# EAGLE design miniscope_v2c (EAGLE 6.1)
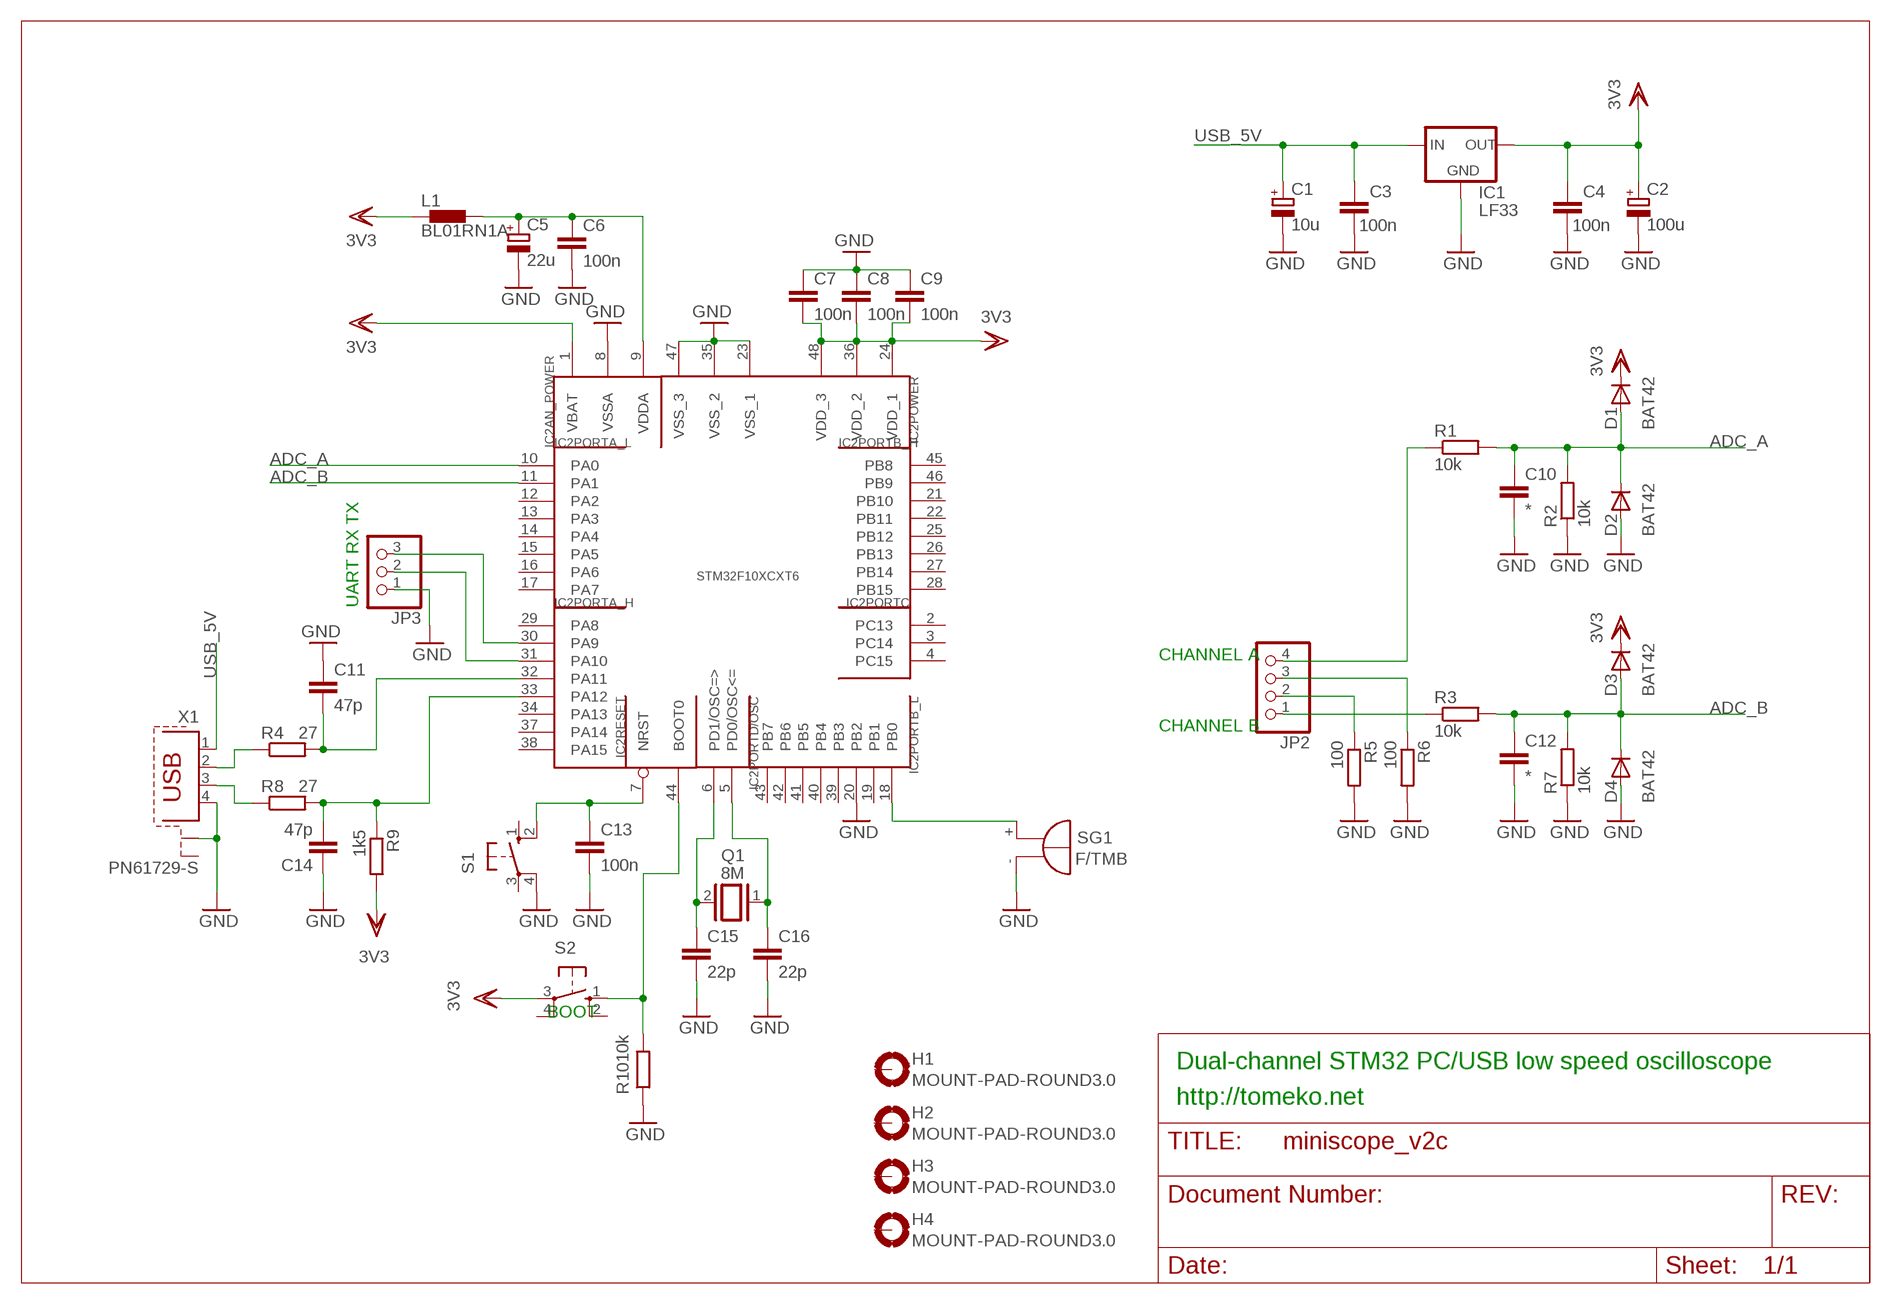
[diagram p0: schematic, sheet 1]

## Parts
C1  10u  CPOL-EUE2.5-5  [E2,5-5]
C2  100u  CPOL-EUE2.5-6  [E2,5-6]
C3  100n  C-EUC0805K  [C0805K]
C4  100n  C-EUC0805K  [C0805K]
C5  22u  CPOL-EUE2.5-5  [E2,5-5]
C6  100n  C-EUC0805K  [C0805K]
C7  100n  C-EUC0805K  [C0805K]
C8  100n  C-EUC0805K  [C0805K]
C9  100n  C-EUC0805K  [C0805K]
C10  *  C-EUC0805K  [C0805K]
C11  47p  C-EUC0805K  [C0805K]
C12  *  C-EUC0805K  [C0805K]
C13  100n  C-EUC0805K  [C0805K]
C14  47p  C-EUC0805K  [C0805K]
C15  22p  C-EUC0805K  [C0805K]
C16  22p  C-EUC0805K  [C0805K]
D1  BAT42  1N4148DO35-7  [DO35-7]
D2  BAT42  1N4148DO35-7  [DO35-7]
D3  BAT42  1N4148DO35-7  [DO35-7]
D4  BAT42  1N4148DO35-7  [DO35-7]
H1  MOUNT-PAD-ROUND3.0  [3,0-PAD]
H2  MOUNT-PAD-ROUND3.0  [3,0-PAD]
H3  MOUNT-PAD-ROUND3.0  [3,0-PAD]
H4  MOUNT-PAD-ROUND3.0  [3,0-PAD]
IC1  LF33  LFXXCV  [DPACK_1]
IC2  STM32F10XCXT6  [TQFP48]
JP2  PINHD-1X4  [1X04]
JP3  PINHD-1X3  [1X03]
L1  BL01RN1A  [BL01RN1A]
Q1  8M  XTAL/S  [QS]
R1  10k  R-R0805  [R0805]
R2  10k  R-R0805  [R0805]
R3  10k  R-R0805  [R0805]
R4  27  R-R0805  [R0805]
R5  100  R-R0805  [R0805]
R6  100  R-R0805  [R0805]
R7  10k  R-R0805  [R0805]
R8  27  R-R0805  [R0805]
R9  1k5  R-R0805  [R0805]
R10  10k  R-R0805  [R0805]
S1  10-XX  [B3F-10XX]
S2  10-XX  [B3F-10XX]
SG1  F/TMB  [F/TMB]
X1  PN61729-S  [PN61729-S]

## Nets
ADC_A: C10.1 D1.A D2.C IC2.10(PORTA_L:PA0) R1.2 R2.2
ADC_B: C12.1 D3.A D4.C IC2.11(PORTA_L:PA1) R3.2 R7.2
GND: C1.- C2.- C3.1 C4.1 C5.- C6.2 C7.1 C8.1 C9.1 C10.2 C11.1 C12.2 C13.2 C14.1 C15.2 C16.2 D2.A D4.A IC1.C(GND) IC2.8(AN_POWER:VSSA) IC2.20(PORTB_L:PB2) IC2.23(POWER:VSS_1) IC2.35(POWER:VSS_2) IC2.47(POWER:VSS_3) JP3.1 R2.1 R5.2 R6.2 R7.1 R10.1 S1.4(P1) SG1.- X1.4 X1.S1
N$1: IC2.44(RESET:BOOT0) R10.2 S2.1(S)
N$2: C5.+ C6.1 IC2.9(AN_POWER:VDDA) L1.2
N$3: JP2.2 R5.1
N$4: C13.1 IC2.7(RESET:NRST) S1.2(S1)
N$5: R4.1 X1.2
N$6: R8.1 X1.3
N$7: C14.2 IC2.33(PORTA_H:PA12) R8.2 R9.1
N$8: C11.2 IC2.32(PORTA_H:PA11) R4.2
N$9: IC2.31(PORTA_H:PA10) JP3.2
N$10: JP2.3 R6.1
N$11: JP2.4 R1.1
N$12: JP2.1 R3.1
N$14: C16.1 IC2.5(PORTD/OSC:PD0/OSC<=) Q1.1
N$15: IC2.18(PORTB_L:PB0) SG1.+
N$16: IC2.30(PORTA_H:PA9) JP3.3
N$37: C15.1 IC2.6(PORTD/OSC:PD1/OSC=>) Q1.2
USB_5V: C1.+ C3.2 IC1.B(IN) X1.1
VDD: C2.+ C4.2 C7.2 C8.2 C9.2 D1.C D3.C IC1.E(OUT) IC2.1(AN_POWER:VBAT) IC2.24(POWER:VDD_1) IC2.36(POWER:VDD_2) IC2.48(POWER:VDD_3) L1.1 R9.2 S2.3(P) ; supply symbol labelled 3V3
Unconnected: H1.B3,0(MOUNT) H2.B3,0(MOUNT) H3.B3,0(MOUNT) H4.B3,0(MOUNT) IC2.2(PORTC:PC13) IC2.3(PORTC:PC14) IC2.4(PORTC:PC15) IC2.12(PORTA_L:PA2) IC2.13(PORTA_L:PA3) IC2.14(PORTA_L:PA4) IC2.15(PORTA_L:PA5) IC2.16(PORTA_L:PA6) IC2.17(PORTA_L:PA7) IC2.19(PORTB_L:PB1) IC2.21(PORTB_H:PB10) IC2.22(PORTB_H:PB11) IC2.25(PORTB_H:PB12) IC2.26(PORTB_H:PB13) IC2.27(PORTB_H:PB14) IC2.28(PORTB_H:PB15) IC2.29(PORTA_H:PA8) IC2.34(PORTA_H:PA13) IC2.37(PORTA_H:PA14) IC2.38(PORTA_H:PA15) IC2.39(PORTB_L:PB3) IC2.40(PORTB_L:PB4) IC2.41(PORTB_L:PB5) IC2.42(PORTB_L:PB6) IC2.43(PORTB_L:PB7) IC2.45(PORTB_H:PB8) IC2.46(PORTB_H:PB9) S1.1(S) S1.3(P) S2.2(S1) S2.4(P1) X1.S2

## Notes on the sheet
- UART RX TX
- CHANNEL A
- CHANNEL B
- BOOT
- Dual-channel STM32 PC/USB low speed oscilloscope
- http://tomeko.net

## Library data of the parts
C1 C2 C5 = resistor:CPOL-EU: POLARIZED CAPACITOR, European symbol
C3 C4 C6-C16 = resistor:C-EU: CAPACITOR, European symbol
D1-D4 = diode:1N4148: DIODE
H1-H4 = holes:MOUNT-PAD-ROUND: MOUNTING PAD, round
IC1 = lf33:LFXXCV: VOLTAGE REGULATOR
IC2 = stm32:STM32F10XCXT6: ST STM32F101/103 48pin LQFP
JP2 = pinhead:PINHD-1X4: PIN HEADER
JP3 = pinhead:PINHD-1X3: PIN HEADER
L1 = inductors:BL0: Noise Suppression Products/EMI Suppression Filters, Lead EMIFIL(R) Inductor Type
Q1 = special:XTAL/S: CRYSTAL
R1-R10 = quantum-sensor:R: Resistor
S1 S2 = switch-omron:10-XX: OMRON SWITCH; MPN: B3F-1000; OC_FARNELL: 176432; OC_NEWARK: 36M3542
SG1 = buzzer:F/TMB: BUZZER; OC_FARNELL: unknown; OC_NEWARK: unknown
X1 = con-berg:PN61729-S: BERG USB connector; OC_FARNELL: unknown; OC_NEWARK: unknown

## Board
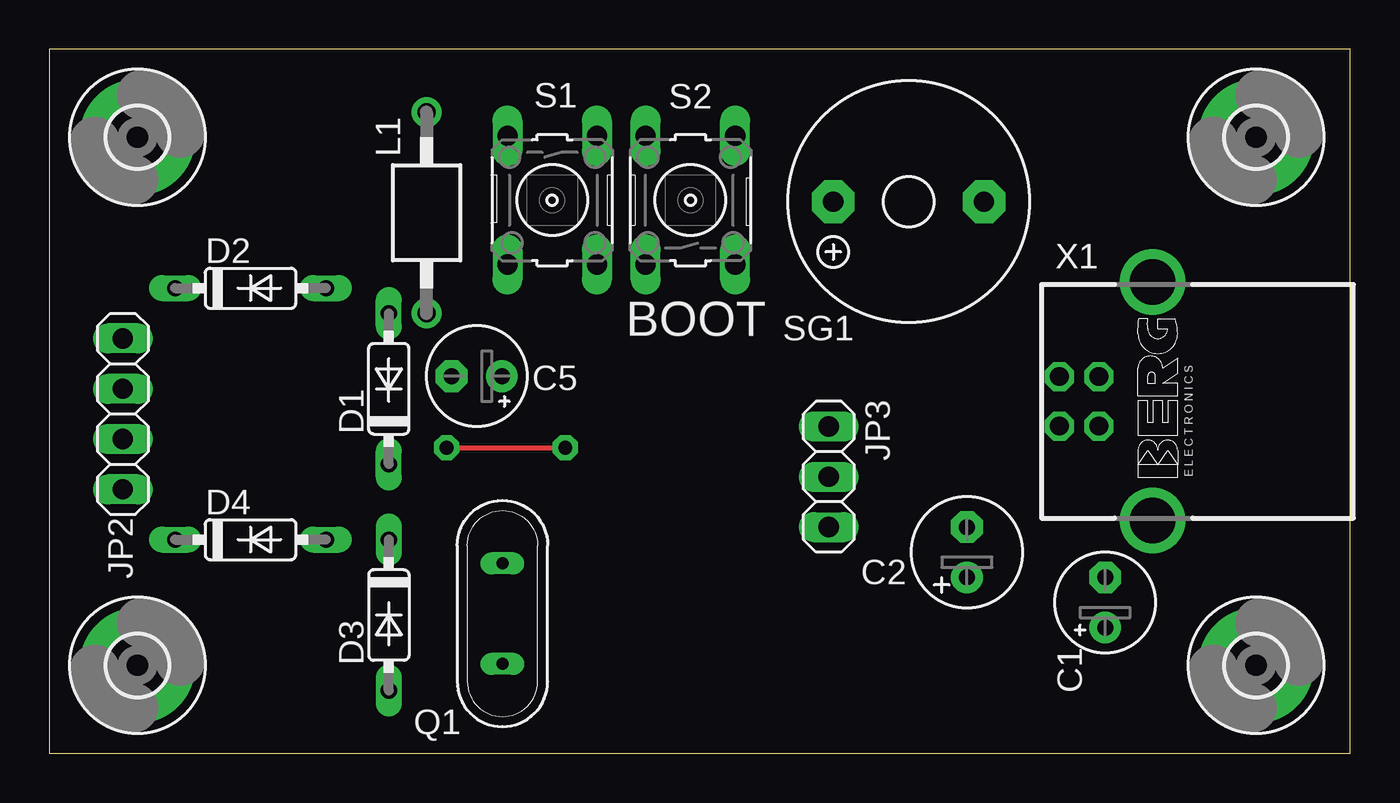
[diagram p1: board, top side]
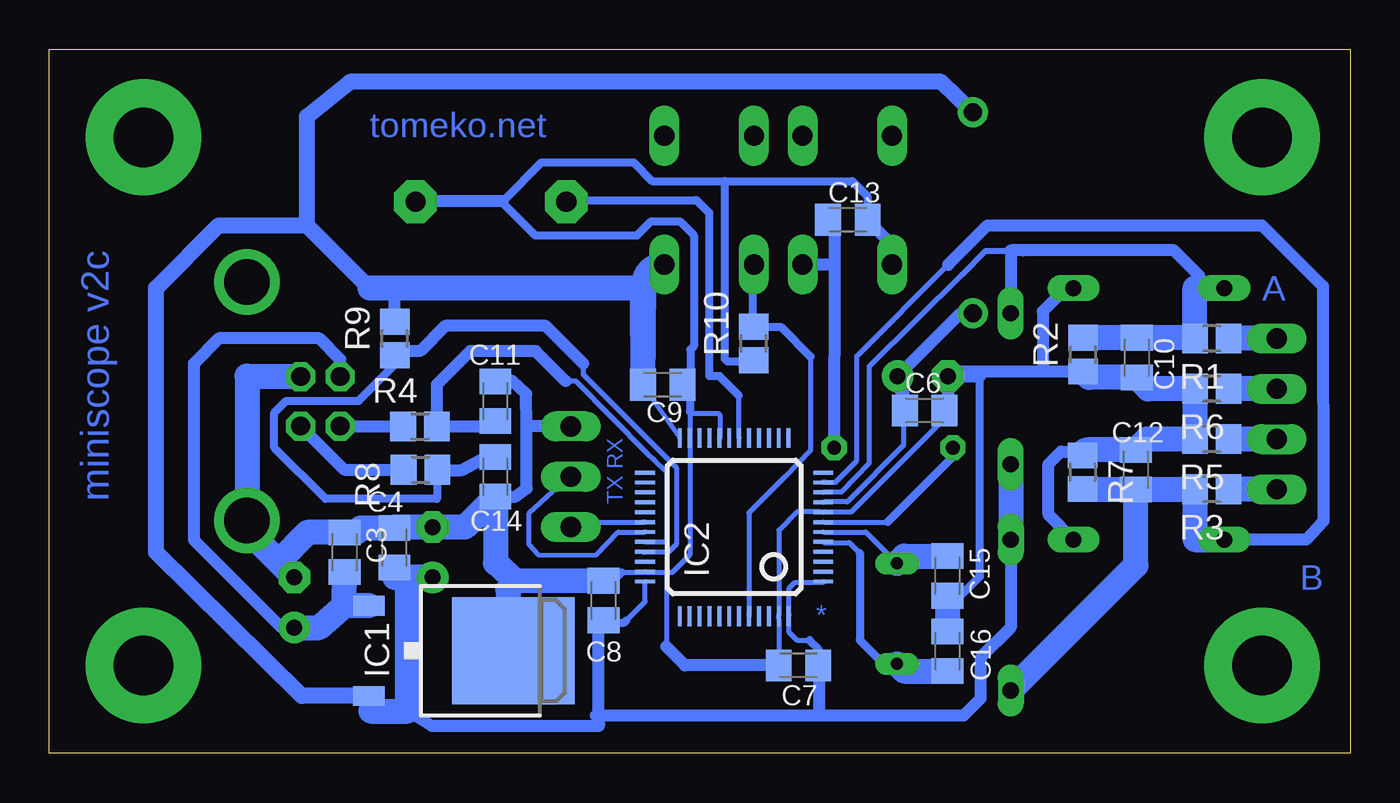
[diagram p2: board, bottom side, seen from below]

Size 65.71 x 35.55 mm. Coordinates in mm from the lower left corner, seen from the top.
Outline: 0,0 65.71,0 65.71,35.55 0,35.55 0,0
Copper layers (1*16): Top 0.035mm / dielectric 1.5mm / Bottom 0.035mm
Design rules: minimum track width 10mil, minimum drill 24mil, track to track 8mil, track to pad 8mil, pad to pad 8mil, via to via 8mil, smd to smd 8mil, copper to edge 40mil, drill to drill 8mil, minimum pad ring 10mil, minimum via ring 8mil, stop-mask expansion 4mil, vias tented up to drill 0mil, thermal gap 10mil

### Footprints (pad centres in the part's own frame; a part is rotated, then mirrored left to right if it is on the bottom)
E2,5-5 = drill 0.813 pad 1.6: + -1.27,0 | drill 0.813 pad 1.6 octagon: - 1.27,0
E2,5-6 = drill 0.813 pad 1.6: + -1.27,0 | drill 0.813 pad 1.6 octagon: - 1.27,0
C0805K = smd 1.3 x 1.6: 1 -1,0; 2 1,0
DO35-7 = drill 0.813 long: A 3.81,0; C -3.81,0
3,0-PAD = drill 3 pad 5.842: B3,0 0,0
DPACK_1 = smd 1 x 1.6: B -2.28,-4.8; E 2.28,-4.8 | smd 5.4 x 6.2: C 0,2.5
TQFP48 = smd 0.2 x 1: 1 -2.75,-4.5; 2 -2.25,-4.5; 3 -1.75,-4.5; 4 -1.25,-4.5; 5 -0.75,-4.5; 6 -0.25,-4.5; 7 0.25,-4.5; 8 0.75,-4.5; 9 1.25,-4.5; 10 1.75,-4.5; 11 2.25,-4.5; 12 2.75,-4.5; 25 2.75,4.5; 26 2.25,4.5; 27 1.75,4.5; 28 1.25,4.5; 29 0.75,4.5; 30 0.25,4.5; 31 -0.25,4.5; 32 -0.75,4.5; 33 -1.25,4.5; 34 -1.75,4.5; 35 -2.25,4.5; 36 -2.75,4.5 | smd 1 x 0.2: 13 4.5,-2.75; 14 4.5,-2.25; 15 4.5,-1.75; 16 4.5,-1.25; 17 4.5,-0.75; 18 4.5,-0.25; 19 4.5,0.25; 20 4.5,0.75; 21 4.5,1.25; 22 4.5,1.75; 23 4.5,2.25; 24 4.5,2.75; 37 -4.5,2.75; 38 -4.5,2.25; 39 -4.5,1.75; 40 -4.5,1.25; 41 -4.5,0.75; 42 -4.5,0.25; 43 -4.5,-0.25; 44 -4.5,-0.75; 45 -4.5,-1.25; 46 -4.5,-1.75; 47 -4.5,-2.25; 48 -4.5,-2.75
1X04 = drill 1.016 long: 1 -3.81,0; 2 -1.27,0; 3 1.27,0; 4 3.81,0
1X03 = drill 1.016 long: 1 -2.54,0; 2 0,0; 3 2.54,0
BL01RN1A = drill 0.9 pad 1.5: 1 -5.08,0; 2 5.08,0
QS = drill 0.61 long: 1 -2.54,0; 2 2.54,0
R0805 = smd 1.3 x 1.5: 1 -0.85,0; 2 0.85,0
B3F-10XX = drill 1.016 long: 1 -3.251,2.261; 2 3.251,2.261; 3 -3.251,-2.261; 4 3.251,-2.261
F/TMB = drill 1.016 pad 2.159 octagon: + 3.81,0; - -3.81,0
PN61729-S = drill 0.95 octagon: 1 1.25,4.71; 2 -1.25,4.71; 3 -1.25,2.71; 4 1.25,2.71 | drill 2.3 pad 2.9: S1 -6.02,0; S2 6.02,0

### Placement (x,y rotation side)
C1  53.34,7.62 90 top
C2  46.35,10.16 90 top
C3  50.8,10.16 270 bottom
C4  48.29,10.39 270 bottom
C5  21.59,19.05 180 top
C6  21.49,17.32 0 bottom
C7  27.86,4.45 0 bottom
C8  37.72,7.72 270 bottom
C9  34.72,18.62 180 bottom
C10  10.77,19.99 270 bottom
C11  43.18,17.78 270 bottom
C12  10.82,14.33 90 bottom
C13  25.37,26.95 0 bottom
C14  43.18,13.97 90 bottom
C15  20.35,8.97 270 bottom
C16  20.35,5.16 90 bottom
D1  17.14,18.41 90 top
D2  10.16,23.5 0 top
D3  17.14,6.99 270 top
D4  10.16,10.79 0 top
H1  60.96,4.45 0 top
H2  60.96,31.11 0 top
H3  4.45,31.11 0 top
H4  4.45,4.45 0 top
IC1  44.78,5.18 270 bottom
IC2  31.11,11.43 90 bottom
JP2  3.71,17.14 90 top
JP3  39.37,13.97 270 top
L1  19.05,27.3 270 top
Q1  22.89,7.06 90 top
R1  6.99,20.95 180 bottom
R2  13.49,20.14 90 bottom
R3  6.99,13.34 180 bottom
R4  46.99,16.51 0 bottom
R5  6.99,15.88 180 bottom
R6  6.99,18.41 180 bottom
R7  13.51,14.2 270 bottom
R8  46.96,14.33 0 bottom
R9  48.26,20.95 90 bottom
R10  30.12,20.7 90 bottom
S1  25.4,27.94 270 top
S2  32.38,27.94 90 top
SG1  43.41,27.86 180 top
X1  55.73,17.78 90 top

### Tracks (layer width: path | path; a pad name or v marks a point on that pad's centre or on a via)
ADC_A
  Bottom 0.254: 19.61,24.18 24.28,19.56 24.28,14.66 25.68,13.21 26.52,13.21 IC2.10 | 17.17,22.25 D1.A
  Bottom 0.305: 19.61,24.18 18.41,25.38 | 18.41,25.38 17.14,25.4 | 18.41,25.38 16.51,25.38
  Bottom 0.406: 16.51,25.38 16.51,25.4
  Bottom 0.61: 7.62,23.5 7.62,24.13 8.89,25.4 16.51,25.4 17.14,25.4 D1.A | 17.17,22.25 17.14,22.28
  Bottom 1.27: D2.C 7.62,23.5 7.83,23.5 R1.2 7.87,20.99 C10.1 R2.2 13.49,20.95 13.34,20.95
ADC_B
  Bottom 0.254: 20.31,24.68 24.92,20.07 24.92,14.78 26.01,13.69 26.49,13.69 26.52,13.72 26.62,13.72 IC2.11 | R3.2 7.82,13.31 8.26,13.34
  Bottom 0.61: 20.3,24.69 20.31,24.68 18.31,26.67 4.45,26.67 1.37,23.6 1.35,11.73 2.21,10.79 D4.C
  Bottom 1.27: C12.1 8.26,13.34 | R3.2 7.83,10.79 D4.C | C12.1 13.49,13.33 R7.2 | D3.A 10.82,9.5 C12.1
GND
  Bottom 0.254: 19.79,7.92 C15.2 19.68,7.95 | 33.25,17.17 31.93,17.17 31.83,17.07 31.83,15.95 IC2.20 | 33.35,17.27 33.25,17.17 | 33.35,18.59 C9.1 | 33.25,17.17 33.35,17.17 33.35,15.95 IC2.23 33.33,15.85 33.33,10.06 34.24,9.14 34.54,9.14 | 36.8,9.14 35.69,9.14 IC2.35 35.56,9.14 34.54,9.14 | C8.1 37.92,8.64 38.1,8.46 38.1,8.26 37.69,8.26 | 13.59,15.09 R7.1 | 34.54,9.14 34.54,5.38 | 28.85,4.37 C7.1 28.85,4.47 28.85,6.81 IC2.47 28.85,7.01 28.85,11.28 27.94,12.19 26.72,12.19 IC2.8 26.52,12.19 25.2,12.19 20.55,16.84 20.55,17.17 20.57,17.14 C6.2 | 55.73,12.29 55.78,12.29 X1.S1 | 42.55,4.47 42.57,4.47 IC1.C | 47.85,11.43 47.85,11.48 C4.1 | 14.02,23.47 D2.A | 31.6,19.91 31.5,19.81 | 30.18,19.81 R10.1 | 33.33,18.69 C9.1 | 47.17,27.89 SG1.- | 42.8,27.79 42.8,27.89 | 33.33,18.8 C9.1
  Bottom 0.406: 33.35,18.59 33.35,17.27 | 31.5,19.81 30.18,19.81 | 36.8,9.14 37.69,8.26 | 42.8,27.89 40.84,29.84 36.2,29.84 35.26,28.91 31.6,28.91 | 42.8,27.79 41.17,26.16 36.02,26.16 35.31,26.87 33.86,26.87 33.15,26.16 33.15,20.57 33.33,20.4 33.33,18.8 33.33,18.64 | 19.68,7.95 18.69,8.94 18.69,19.05 | 31.6,28.91 31.6,19.91 | 31.6,28.91 25.15,28.91 24.38,28.14 24.38,27 24.41,26.98 24.4,26.98 C13.2
  Bottom 0.61: C14.1 42.17,12.97 41.6,13.39 41.6,16.51 | 41.6,16.51 41.63,18.16 42.32,18.8 43.18,19.05 C11.1 | JP3.1 41.6,16.51 | 28.85,4.37 C7.1 33.6,4.45 34.54,5.38 | D4.A 15.24,12.06 15.24,14.61 14.61,15.24 13.34,15.24 13.51,15.06 R7.1 | 42.8,27.89 47.17,27.89 | C5.- 18.69,19.05 | C5.- 20.08,19.29 15.37,19.29 | 15.37,19.29 R2.1 13.34,19.14 13.34,19.05 | D2.A 14.35,23.5 15.52,22.33 15.52,19.45 15.37,19.29 | C5.- 20.32,17.41 C6.2 20.32,17.14 | S1.4 23.14,25.68 24.38,26.91 C13.2
  Bottom 1.27: R2.1 13.19,18.99 C10.2 10.2,18.41 R6.2 R5.2 10.27,15.88 C12.2 13.24,15.33 arc-90 R7.1 | C16.2 C15.2 arc90 20.32,7.94 20.32,7.62 | 55.73,11.91 55.73,12.29 55.73,19.05 55.71,19.03 X1.4 | X1.S1 55.73,11.28 54.14,9.69 | 54.14,9.69 C1.- | 54.14,9.69 52.67,11.16 C3.1 50.19,11.18 49.98,11.39 C4.1 | 48.26,11.43 47.85,11.43 C2.- 44.72,11.43 C14.1 43.18,9.62 42.16,8.7 | C8.1 42.16,8.7 | 42.16,8.7 42.55,8.26 42.55,4.47 42.55,4.45
N$1
  Bottom 0.254: 27.25,20.04 27.25,15.32 28.55,13.97 30.38,12.14 30.38,7.01 IC2.44 | 30.07,21.54 R10.2 30.18,21.64 | 30.18,24.69 S2.1
  Bottom 0.406: 27.25,20.04 28.75,21.54 30.07,21.54 | 30.18,21.64 30.18,24.69
N$2
  Bottom 0.254: IC2.9 26.52,12.7 25.4,12.7 22.55,15.57 22.55,16.66 C6.1 22.55,16.76 | 19.1,22.35 19.1,22.86 L1.2 | C5.+ 22.86,18.59
  Bottom 0.61: 22.55,16.76 22.55,18.19 22.76,18.39 C5.+ 19.68,22.23 L1.2
N$3
  Bottom 1.27: JP2.2 R5.1
N$4  (via drill 0.7 pad 1.27)
  Top 0.254: v20.07,15.44 v26.06,15.44
  Bottom 0.254: IC2.7 23.37,11.68
  Bottom 0.406: 23.37,11.68 20.07,14.99 v20.07,15.44
  Bottom 0.61: v26.06,15.44 26.04,24.69 | 26.04,24.69 S1.2 | 26.04,24.69 26.04,26.61 C13.1
N$5
  Bottom 0.254: R4.1 47.85,16.56 47.62,16.53
  Bottom 0.61: X1.2 47.62,16.53 47.62,16.51
N$6
  Bottom 0.61: X1.3 50.81,14.33 R8.1
N$7
  Bottom 0.254: 35.69,10.13 IC2.33 35.56,10.16 34.44,10.16 34.04,10.57 34.04,14.43 38.73,19.13 38.73,19.68 | C14.2 43.18,14.94 43.31,15.17 | 48.26,20.12 R9.1 48.36,20.12 | 46.13,14.02 R8.2
  Bottom 0.406: 46.13,14.02 46.13,12.85 51.77,12.85 54.36,15.44 54.36,17.2 53.75,17.8 50.09,17.8 48.26,19.63 R9.1
  Bottom 0.61: R8.2 46.12,14.3 44.88,14.3 43.31,15.17 43.18,15.24 | 38.73,19.68 40.64,21.59 45.72,21.59 46.99,20.32 48.26,20.32 48.26,20.12
N$8
  Bottom 0.254: IC2.32 35.56,10.67 34.65,10.67 34.54,10.77 34.54,14.22 35.15,14.83 35.53,15.19 39.12,18.8 39.62,18.8 | 46.13,16.76 R4.2
  Bottom 0.61: C11.2 43.18,16.51 R4.2 46.14,18.63 44.45,20.32 41.15,20.32 39.62,18.8
N$9
  Bottom 0.254: IC2.31 35.66,11.18 36.98,11.18 38.1,10.01 41.02,10.03 41.5,10.57 41.5,12.09 39.42,14.02 JP3.2
N$10
  Bottom 1.27: JP2.3 R6.1
N$11
  Bottom 1.27: JP2.4 R1.1
N$12
  Bottom 1.27: JP2.1 R3.1
N$14
  Bottom 0.254: IC2.5 26.58,10.64 25.3,10.64 24.77,10.11
  Bottom 0.406: 24.77,10.11 24.77,5.71 23.57,4.52 Q1.1
  Bottom 1.27: Q1.1 22.52,4.16 C16.1
N$15
  Bottom 0.254: 30.89,18.09 30.89,15.95 IC2.18 | SG1.+ 39.62,27.84 39.52,27.84
  Bottom 0.406: 39.52,27.84 39.42,27.94 33.02,27.94 32.38,27.3 32.38,19.05 31.85,19.05 30.89,18.09
N$16
  Bottom 0.254: 39.12,11.68 JP3.3 39.01,11.68 35.76,11.68 IC2.30 35.66,11.68
N$37
  Bottom 0.254: IC2.6 24.46,11.18 Q1.2 | Q1.2 22.86,9.58 22.86,9.53 22.89,9.55 Q1.2
  Bottom 1.27: Q1.2 22.52,9.97 C15.1
USB_5V
  Bottom 0.61: X1.1 51.02,19.9 52.07,20.95 57.15,20.95 58.42,19.68 58.42,10.79 53.98,6.35 C1.+
  Bottom 1.27: IC1.B 50.83,7.46 | 50.83,7.46 C3.2 | C1.+ 52.09,6.35 50.83,7.46
VDD
  Bottom 0.254: 27.3,5.71 27.94,5.71 28.37,6.15 28.37,6.92 IC2.48 28.35,7.01 28.35,8.33 28.04,8.64 26.62,8.64 IC2.1 | 37.9,6.6 C8.2 38,6.6 | 48.36,21.84 R9.2 | 26.82,4.37 C7.2 | 52.53,27.03 52.7,26.67 | 49.48,2.13 IC1.E | 17.17,10.87 D3.C | 17.17,14.53 D1.C | IC2.24 35.75,18.62 | 36.58,6.71 35.62,7.67 IC2.36
  Bottom 0.406: 27.3,5.71 26.86,5.27 C7.2 | 36.58,6.71 36.68,6.6 37.9,6.6
  Bottom 0.61: 38,6.6 38,1.91 | 38,1.91 37.95,1.37 46.38,1.37 47.62,2.13 | 26.82,4.37 26.82,1.91 | 26.82,1.91 38,1.91 | 38.1,1.91 38,1.91 | 17.17,10.87 17.14,10.85 17.14,6.35 18.67,4.83 18.67,2.77 19.53,1.91 26.82,1.91 | 48.26,22.23 48.26,23.5
  Bottom 0.813: IC1.E 52.97,2.9 60.33,10.16 60.33,23.5 57.15,26.67 52.7,26.67 | 52.7,26.67 49.53,23.5 | 48.26,22.23 R9.2 48.26,21.59 | L1.1 20.65,33.91 50.52,33.91 52.7,32.16 52.7,26.67
  Bottom 1.27: C2.+ 47.62,8.89 | 49.48,2.13 47.62,2.13 47.62,8.89 | 47.62,8.89 48.26,8.89 C4.2 | 17.17,14.53 17.14,14.5 D3.C | C9.2 35.67,23.69 arc90 S2.3 | C9.2 35.75,23.5 48.26,23.5 49.53,23.5 | C9.2 35.75,18.62

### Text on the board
Bottom: tomeko.net | miniscope v2c | A | TX RX | B | *
tNames: BOOT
